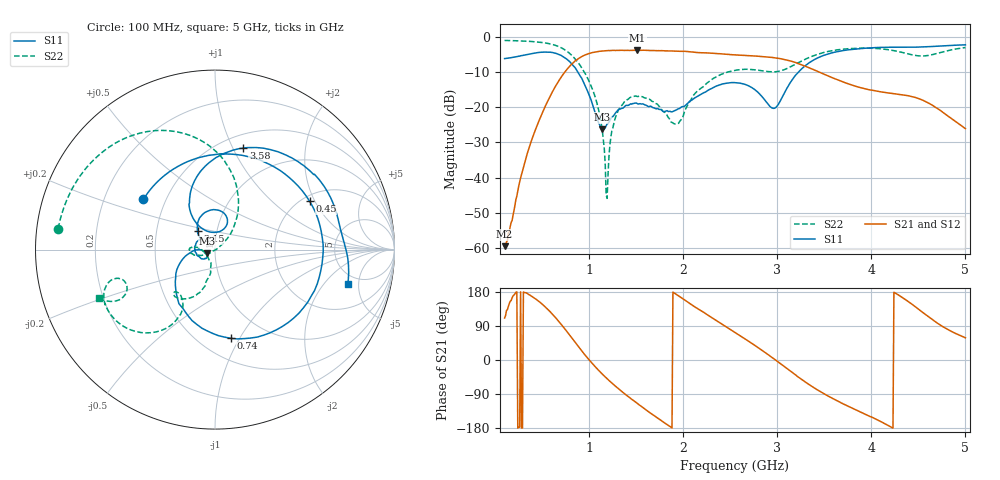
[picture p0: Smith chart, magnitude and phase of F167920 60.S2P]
!  2-Port S-parameters saved by WinCal
! VAR MeasName=S-Parameters (CALIBRATED_DATA) read from VNA (N5242A)
! VAR MeasDate=2016-11-22 9:58:30
! VAR NAME=F167920 60
! VAR FILENAME=F167920 60.S2P
! VAR DATE=2016-11-22 9:58:30
! VAR PHYS_PORTS=1,2
# Hz S DB R 50
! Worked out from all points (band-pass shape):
!   491 points, 100 MHz to 5 GHz, reference 50 ohm
!   highest |S21| = -3.87 dB at 1.51 GHz (marker M1); lowest = -59.5 dB at 100 MHz (marker M2)
!   |S21| within 3 dB of the highest: 851.2 MHz to 3.133 GHz (2.282 GHz wide, 115 % of centre)
!   lowest |S11| = -26.3 dB at 1.14 GHz (marker M3), VSWR 1.10, Z = 45.7 - j1.85 ohm
!   |S11| at or under -10 dB: 876.8 MHz to 3.227 GHz (2.35 GHz wide, 115 % of centre)
!   |S22| runs from -45.9 to -1.1 dB; largest |S21 - S12| = 0.0015
!   S11 on the Smith chart (normalised r, x): 100 MHz: 0.37, +0.28; 450 MHz: 2.19, +1.82; 740 MHz: 0.70, -0.92; 2.15 GHz: 0.81, +0.17; 3.58 GHz: 0.64, +1.10; 5 GHz: 4.02, -3.66
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1e8  -6.25 144.9  -59.46 110.9  -59.46 111.4  -1.10 172.4
2.9e8  -5.36 80.4  -38.10 -179.7  -38.11 -180.0  -1.25 157.4
4.5e8  -4.55 27.1  -24.93 157.4  -24.94 157.5  -1.53 142.5
5.9e8  -4.44 -22.4  -16.60 125.9  -16.59 125.9  -2.11 125.7
7.4e8  -5.99 -79.9  -10.08 82.3  -10.07 82.3  -3.74 102.2
9.2e8  -11.81 -148.2  -5.65 24.3  -5.64 24.4  -8.89 70.1
1.06e9  -21.39 -179.2  -4.40 -16.9  -4.40 -16.9  -16.88 47.9
1.14e9  -26.28 -155.5  -4.09 -37.5  -4.09 -37.4  -26.87 36.0
1.19e9  -24.75 -138.0  -3.99 -49.3  -3.99 -49.3  -45.90 -127.3
1.24e9  -22.72 -136.8  -3.93 -60.5  -3.93 -60.5  -26.80 -151.4
1.29e9  -21.34 -142.6  -3.92 -71.5  -3.92 -71.5  -22.14 -156.1
1.51e9  -19.00 169.0  -3.87 -114.4  -3.86 -114.4  -17.00 -179.6
1.74e9  -20.65 137.6  -3.99 -155.4  -3.99 -155.4  -19.71 173.0
1.93e9  -20.76 139.7  -4.15 172.4  -4.15 172.4  -24.71 -140.6
2.15e9  -16.99 133.4  -4.53 135.9  -4.53 135.9  -15.45 -104.2
2.55e9  -13.07 89.2  -5.18 72.6  -5.20 72.6  -9.57 -124.0
2.97e9  -20.32 95.7  -6.01 2.0  -6.02 2.0  -10.00 -128.7
3.37e9  -6.89 99.1  -9.20 -70.1  -9.23 -70.0  -5.58 -122.5
3.58e9  -4.62 74.3  -11.63 -100.6  -11.66 -100.4  -4.01 -133.4
4.19e9  -3.02 24.3  -16.01 -174.2  -16.05 -173.9  -3.76 -160.7
4.6e9  -2.88 4.0  -18.73 115.4  -18.76 115.7  -5.38 -155.6
5e9  -2.34 -14.4  -26.12 58.6  -26.10 59.1  -3.11 -157.1
